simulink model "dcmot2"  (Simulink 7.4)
settings: Solver=ode45  StartTime=0.0  StopTime=4  MaxStep=0.005  RelTol=1e-3

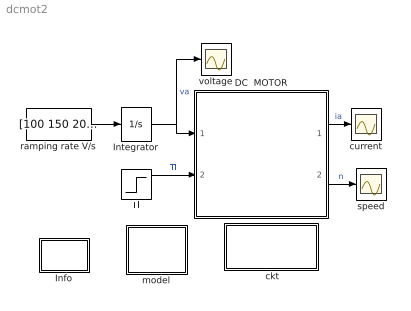
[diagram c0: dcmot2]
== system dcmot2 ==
  " ckt" : Subsystem
  DC  MOTOR : Subsystem  mask{Ra=0.70, La=0.03, J=0.60, Bm=1e-3, K=2}
      mask prompts: Ra "Armature resistance [ohm]"; La "Armature inductance [H]"; J "Moment of inertia [Kg.m^2]"; Bm "Frictional torque cefficient"; K "Electromechanical coupling coefficient [N.m/A]"
      mask help: Dynamic model of a dc motor
  Info : Subsystem
  Integrator : Integrator  LimitOutput=on  UpperSaturationLimit=240  LowerSaturationLimit=-240
  Tl : Step  Time=3  Before=4  After=30  SampleTime=0
  current : Scope
  model : Subsystem
  ramping rate V/s : Constant  Value=[100 150 200]  OutDataType=sfix(16)  OutScaling=2^0
  speed : Scope
  voltage : Scope
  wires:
  Tl/1 -> DC  MOTOR/2(Tl)  "Tl"
  DC  MOTOR/1(ia) -> current/1  "ia"
  DC  MOTOR/2(n) -> speed/1  "n"
  Integrator/1 -> DC  MOTOR/1(va), voltage/1  "va"
  ramping rate V/s/1 -> Integrator/1

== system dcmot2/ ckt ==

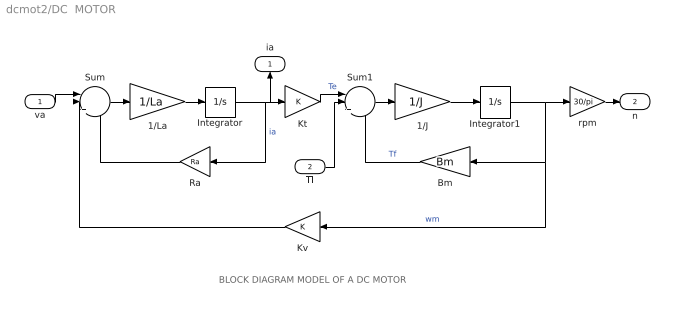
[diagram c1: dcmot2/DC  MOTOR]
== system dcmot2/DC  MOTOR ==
  note: BLOCK DIAGRAM MODEL OF A DC MOTOR
  va : Inport  OutDataType=sfix(16)  OutScaling=2^0
  Tl : Inport  Port=2  OutDataType=sfix(16)  OutScaling=2^0
  1/J : Gain  Gain=1/J  ParameterDataType=sfix(16)  ParameterScaling=2^0  OutDataType=sfix(16)  OutScaling=2^0
  1/La : Gain  Gain=1/La  ParameterDataType=sfix(16)  ParameterScaling=2^0  OutDataType=sfix(16)  OutScaling=2^0
  Bm : Gain  Gain=Bm  ParameterDataType=sfix(16)  ParameterScaling=2^0  OutDataType=sfix(16)  OutScaling=2^0
  Integrator : Integrator
  Integrator1 : Integrator
  Kt : Gain  Gain=K  ParameterDataType=sfix(16)  ParameterScaling=2^0  OutDataType=sfix(16)  OutScaling=2^0
  Kv : Gain  Gain=K  ParameterDataType=sfix(16)  ParameterScaling=2^0  OutDataType=sfix(16)  OutScaling=2^0
  Ra : Gain  Gain=Ra  ParameterDataType=sfix(16)  ParameterScaling=2^0  OutDataType=sfix(16)  OutScaling=2^0
  Sum : Sum  Inputs=||+--  OutDataType=sfix(16)  OutScaling=2^0
  Sum1 : Sum  Inputs=||+--  OutDataType=sfix(16)  OutScaling=2^0
  rpm : Gain  Gain=30/pi  ParameterDataType=sfix(16)  ParameterScaling=2^0  OutDataType=sfix(16)  OutScaling=2^0
  ia : Outport
  n : Outport  Port=2
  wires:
  Kv/1 -> Sum/2
  Ra/1 -> Sum/3
  Kt/1 -> Sum1/1  "Te"
  Bm/1 -> Sum1/3  "Tf"
  Sum/1 -> 1/La/1
  1/La/1 -> Integrator/1
  Integrator/1 -> Ra/1, Kt/1, ia/1  "ia"
  Sum1/1 -> 1/J/1
  1/J/1 -> Integrator1/1
  va/1 -> Sum/1
  Tl/1 -> Sum1/2
  Integrator1/1 -> Bm/1, Kv/1, rpm/1  "wm"
  rpm/1 -> n/1

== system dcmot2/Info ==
  note: This demo simulates the ramp start of a DC motor with constant field or pm excitation (5 hp 240V 1200 rpm) rated torque Tr = 30 N.m

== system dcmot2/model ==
  note: Mathematical model of the dc machine
  note: Electrical system equation: va = Ra.ia + La.dia/dt + ea where ea = K.wm Mechanical system equation: Te = J.dwm/dt + Tl.signum(wm) + f(wm) where Te = K.ia
